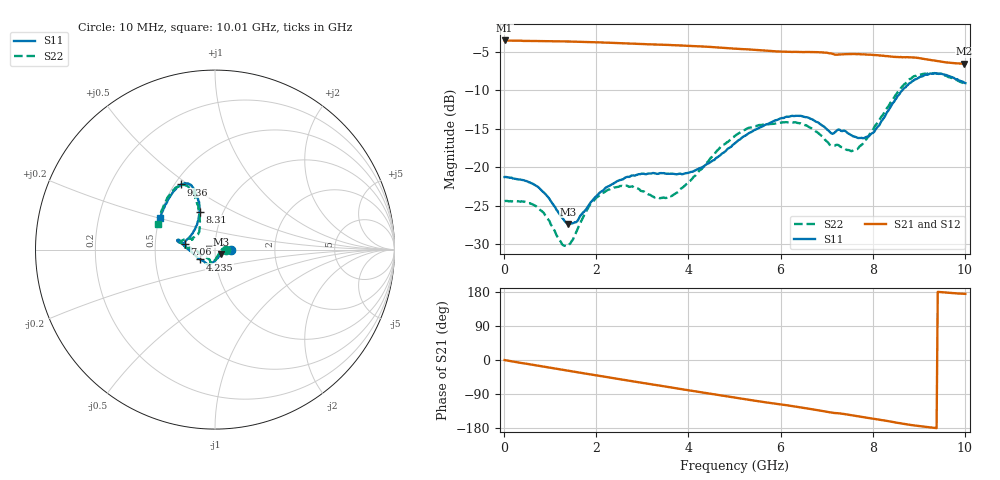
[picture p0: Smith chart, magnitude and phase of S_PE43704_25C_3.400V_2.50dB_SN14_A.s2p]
! Device ID: PE43704
! Dir: z:\PE43704\PE43704_Char_1_20130516\PE43704\AMB\3p400V\2p50dB
! Serial: 14
! Insertion: A
! Impedance: 50 ohm
! Temp: Amb
! VDD: 3.400V
! Attenuation Step: 2.50dB
! IDD: 1.141072e-01mA
#  Hz  S  RI  R  50
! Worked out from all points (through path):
!   401 points, 10 MHz to 10.01 GHz, reference 50 ohm
!   highest |S21| = -3.52 dB at 10 MHz (marker M1); lowest = -6.5 dB at 9.985 GHz (marker M2)
!   group delay of S21, straight-line fit = 52.8 ps
!   lowest |S11| = -27.4 dB at 1.385 GHz (marker M3), VSWR 1.09, Z = 53.6 - j2.62 ohm
!   |S11| at or under -10 dB: start of sweep to 8.641 GHz
!   |S22| runs from -30.3 to -7.8 dB; largest |S21 - S12| = 0.005
!   S11 on the Smith chart (normalised r, x): 10 MHz: 1.19, +0.00; 4.235 GHz: 0.84, -0.09; 7.06 GHz: 0.71, +0.05; 8.31 GHz: 0.77, +0.35; 9.36 GHz: 0.54, +0.47; 10.01 GHz: 0.50, +0.20
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1e7  0.0865 6.54e-05  0.6672 -0.00269  0.6674 -0.00268  0.0603 0.000332
6.85e8  0.075 0.013  0.6421 -0.1598  0.642 -0.1596  0.0534 0.0169
1.26e9  0.0446 -0.0144  0.5936 -0.2849  0.5936 -0.2846  0.0298 -0.0103
1.385e9  0.0353 -0.0244  0.5792 -0.31  0.5794 -0.31  0.0235 -0.0201
1.685e9  0.0152 -0.0472  0.5405 -0.3681  0.5405 -0.3678  0.0086 -0.0445
1.985e9  -0.00224 -0.0643  0.4954 -0.4198  0.4954 -0.4197  -0.00326 -0.0627
2.385e9  -0.0198 -0.0763  0.4284 -0.4795  0.4285 -0.4793  -0.0168 -0.0719
3.36e9  -0.0409 -0.0815  0.242 -0.578  0.2427 -0.5776  -0.0331 -0.0539
3.735e9  -0.0541 -0.072  0.1646 -0.5987  0.1655 -0.5985  -0.0545 -0.0408
4.235e9  -0.0819 -0.0549  0.059 -0.6079  0.0598 -0.6078  -0.094 -0.0154
5.01e9  -0.1434 -0.00355  -0.0954 -0.5822  -0.0951 -0.5824  -0.1596 0.0104
5.985e9  -0.2 0.0534  -0.2562 -0.5044  -0.2536 -0.5049  -0.1912 0.038
6.685e9  -0.201 0.0405  -0.361 -0.4292  -0.3613 -0.4286  -0.169 0.0562
7.06e9  -0.1678 0.0319  -0.4079 -0.3693  -0.4083 -0.3712  -0.1287 0.0563
7.66e9  -0.1367 0.0746  -0.4611 -0.286  -0.461 -0.2873  -0.0891 0.0961
7.985e9  -0.1071 0.1275  -0.486 -0.2315  -0.4858 -0.2332  -0.0849 0.1505
8.31e9  -0.086 0.2112  -0.4988 -0.1735  -0.4976 -0.1751  -0.0926 0.2249
8.36e9  -0.0852 0.2236  -0.4995 -0.1629  -0.4996 -0.1653  -0.0931 0.2383
8.835e9  -0.1178 0.3366  -0.5122 -0.0756  -0.5089 -0.0779  -0.1472 0.3477
9.36e9  -0.1879 0.363  -0.4925 -0.00376  -0.4928 -0.00233  -0.2214 0.3436
9.985e9  -0.301 0.1863  -0.4687 0.044  -0.4702 0.0461  -0.3132 0.1523
1.001e10  -0.3062 0.1742  -0.4698 0.0452  -0.4724 0.0462  -0.3161 0.1426
